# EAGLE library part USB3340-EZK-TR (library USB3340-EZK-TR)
Microchip USB3340-EZK-TR, USB Transceiver, USB 2.0 at 480Mbit/s, 5.5 V, 32-Pin QFN Source: Datasheet
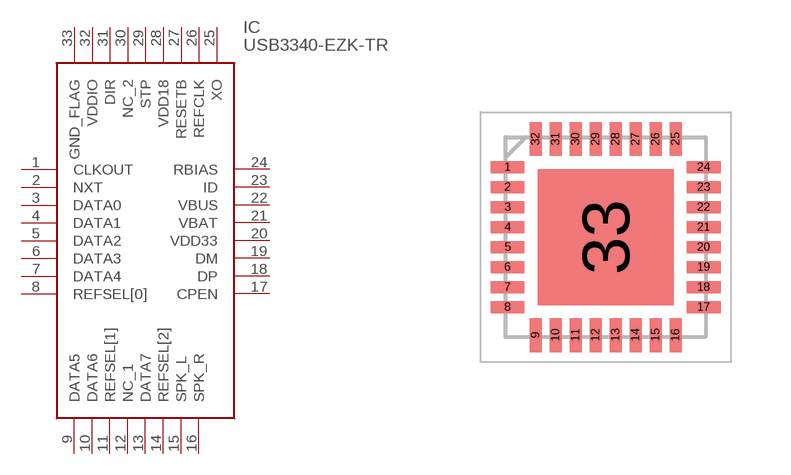
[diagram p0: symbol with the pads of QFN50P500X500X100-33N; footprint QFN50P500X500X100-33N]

Designator prefix IC

## USB3340-EZK-TR (Description: Microchip USB3340-EZK-TR, USB Transceiver, USB 2.0 at 480Mbit/s, 5.5 V, 32-Pin QFN; Height: 1mm; Manufacturer_Name: Microchip; Manufacturer_Part_Number: USB3340-EZK-TR; Mouser_Part_Number: 886-USB3340-EZK-TR; Mouser_Price-Stock: https://www.mouser.co.uk/ProductDetail/Microchip-Technology/USB3340-EZK-TR?qs=pA5MXup5wxES2TIeidc1qQ%3D%3D)  [QFN50P500X500X100-33N]
1  CLKOUT
2  NXT
3  DATA0
4  DATA1
5  DATA2
6  DATA3
7  DATA4
8  REFSEL[0]
9  DATA5
10  DATA6
11  REFSEL[1]
12  NC_1
13  DATA7
14  REFSEL[2]
15  SPK_L
16  SPK_R
17  CPEN
18  DP
19  DM
20  VDD33
21  VBAT
22  VBUS
23  ID
24  RBIAS
25  XO
26  REFCLK
27  RESETB
28  VDD18
29  STP
30  NC_2
31  DIR
32  VDDIO
33  GND_FLAG

## Footprint QFN50P500X500X100-33N (pad centres in mm)
32 Pin QFN
smd 0.85 x 0.3: 1 -2.45,1.75; 2 -2.45,1.25; 3 -2.45,0.75; 4 -2.45,0.25; 5 -2.45,-0.25; 6 -2.45,-0.75; 7 -2.45,-1.25; 8 -2.45,-1.75; 17 2.45,-1.75; 18 2.45,-1.25; 19 2.45,-0.75; 20 2.45,-0.25; 21 2.45,0.25; 22 2.45,0.75; 23 2.45,1.25; 24 2.45,1.75
smd 0.3 x 0.85: 9 -1.75,-2.45; 10 -1.25,-2.45; 11 -0.75,-2.45; 12 -0.25,-2.45; 13 0.25,-2.45; 14 0.75,-2.45; 15 1.25,-2.45; 16 1.75,-2.45; 25 1.75,2.45; 26 1.25,2.45; 27 0.75,2.45; 28 0.25,2.45; 29 -0.25,2.45; 30 -0.75,2.45; 31 -1.25,2.45; 32 -1.75,2.45
smd 3.4 x 3.4: 33 0,0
